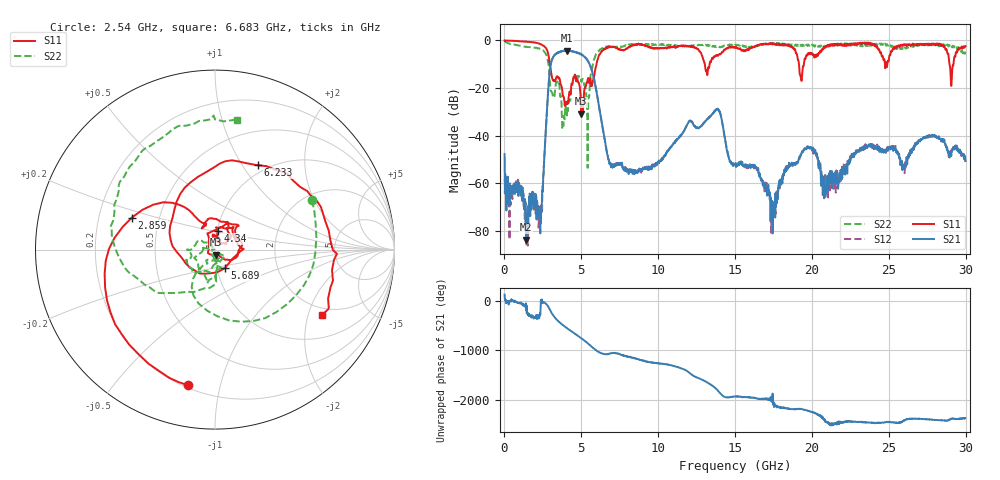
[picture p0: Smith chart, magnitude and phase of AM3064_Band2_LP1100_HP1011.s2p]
# Hz S DB R 50.0
!freq dBS11 angS11 dBS21 angS21 dBS12 angS12 dBS22 angS22
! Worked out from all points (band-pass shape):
!   1600 points, 10 MHz to 29.98 GHz, reference 50 ohm
!   highest |S21| = -4.25 dB at 4.077 GHz (marker M1); lowest = -83.6 dB at 1.416 GHz (marker M2)
!   |S21| within 3 dB of the highest: 3.147 GHz to 5.267 GHz (2.12 GHz wide, 50.4 % of centre)
!   lowest |S11| = -30.8 dB at 4.996 GHz (marker M3), VSWR 1.06, Z = 50.6 - j2.85 ohm
!   |S11| at or under -10 dB: 2.955 GHz to 5.987 GHz (3.031 GHz wide, 67.8 % of centre); 13.03 GHz to 13.34 GHz (309 MHz wide, 2.34 % of centre); 19.16 GHz to 19.48 GHz (319.8 MHz wide, 1.66 % of centre)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
!   |S22| runs from -53.5 to -0.3 dB; largest |S21 - S12| = 0.019
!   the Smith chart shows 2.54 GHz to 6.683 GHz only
!   S11 on the Smith chart (normalised r, x): 2.54 GHz: 0.21, -0.80; 2.859 GHz: 0.35, +0.16; 4.34 GHz: 1.01, +0.21; 5.689 GHz: 1.09, -0.22; 6.233 GHz: 0.90, +1.17; 6.683 GHz: 1.72, -2.45
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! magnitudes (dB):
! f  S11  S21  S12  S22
! 10 MHz  0.0  -47.7  -58.3  -0.3
! 1.416 GHz  -0.5  -83.6  -73.5  -2.7
! 2.297 GHz  -1.5  -71.5  -77.7  -3.5
! 2.54 GHz  -2.3  -56.2  -56.3  -4.3
! 2.859 GHz  -6.1  -19.6  -19.6  -10.1
! 4.077 GHz  -26.7  -4.3  -4.4  -29.7
! 4.34 GHz  -19.5  -4.6  -4.5  -20.4
! 4.996 GHz  -30.8  -5.9  -5.8  -17.3
! 5.015 GHz  -29.8  -6.0  -5.9  -17.4
! 5.408 GHz  -16.6  -8.4  -8.3  -53.5
! 5.689 GHz  -18.7  -12.6  -12.7  -12.3
! 6.233 GHz  -5.6  -30.7  -30.7  -3.7
! 6.683 GHz  -3.1  -47.8  -47.7  -2.7
! 10 GHz  -3.4  -51.2  -51.0  -1.8
! 13.82 GHz  -6.2  -28.8  -28.8  -2.6
! 15 GHz  -2.8  -52.3  -52.4  -1.8
! 16.35 GHz  -2.4  -53.4  -53.2  -2.5
! 17.46 GHz  -1.2  -79.2  -74.1  -1.4
! 19.99 GHz  -5.4  -45.2  -45.2  -1.8
! 20.85 GHz  -2.9  -62.3  -56.5  -2.5
! 25 GHz  -8.5  -45.5  -45.8  -1.7
! 29.98 GHz  -2.4  -50.6  -50.9  -4.7
